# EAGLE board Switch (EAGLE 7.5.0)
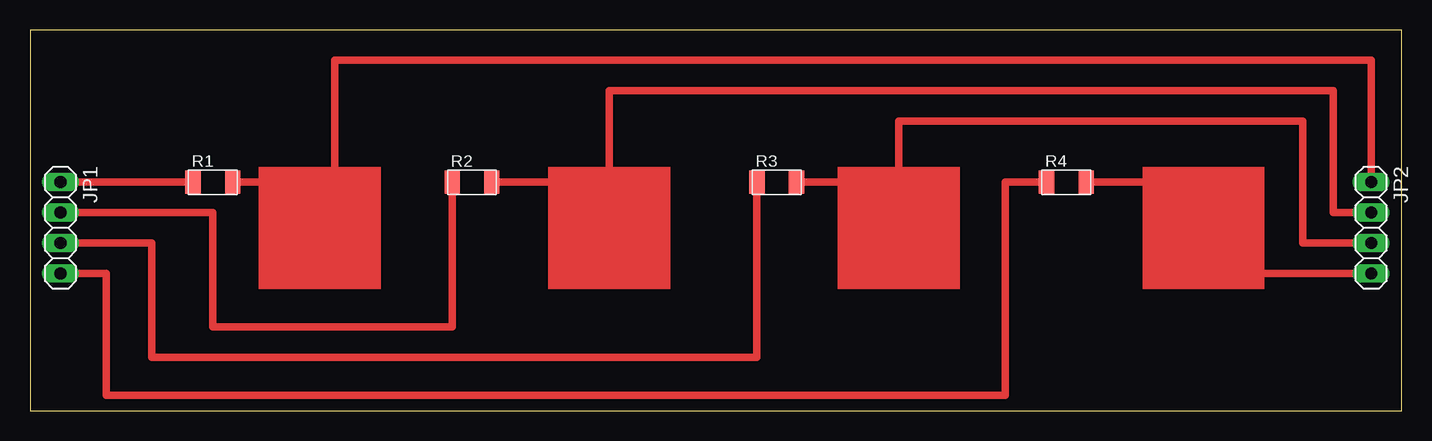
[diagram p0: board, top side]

Size 114.3 x 31.75 mm. Coordinates in mm from the lower left corner, seen from the top.
Outline: 0,0 114.3,0 114.3,31.75 0,31.75 0,0
Copper layers (1*16): Top 0.035mm / dielectric 1.5mm / Bottom 0.035mm
Design rules "default": minimum track width 10mil, minimum drill 24mil, track to track 8mil, track to pad 8mil, pad to pad 8mil, via to via 8mil, smd to smd 8mil, copper to edge 40mil, drill to drill 8mil, minimum pad ring 10mil, minimum via ring 8mil, stop-mask expansion 4mil, vias tented up to drill 0mil, thermal gap 10mil

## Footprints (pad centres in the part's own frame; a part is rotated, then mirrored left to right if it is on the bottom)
1X04 = drill 1.016 long: 1 -3.81,0; 2 -1.27,0; 3 1.27,0; 4 3.81,0
R1206FAB = smd 1.27 x 1.905: 1 -1.651,0; 2 1.651,0

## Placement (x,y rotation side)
JP1  [1X04]  2.54,15.24 270 top
JP2  [1X04]  111.76,15.24 270 top
R1  [R1206FAB]  15.24,19.05 0 top
R2  [R1206FAB]  36.83,19.05 0 top
R3  [R1206FAB]  62.23,19.05 0 top
R4  [R1206FAB]  86.36,19.05 0 top

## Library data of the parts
JP1 JP2 = pinhead
R1-R4 = fab

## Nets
N$1: JP1.1 R1.1
N$3: JP1.2 R2.1
N$4: JP2.2 R2.2
N$5: JP1.3 R3.1
N$6: JP2.3 R3.2
N$7: JP1.4 R4.1
N$8: JP2.4 R4.2
N$9: JP2.1 R1.2

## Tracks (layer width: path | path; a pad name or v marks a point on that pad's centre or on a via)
N$1
  Top 0.61: JP1.1 R1.1
N$3
  Top 0.61: JP1.2 15.24,16.51 15.24,6.99 35.18,6.99 R2.1
N$4
  Top 0.61: R2.2 48.26,19.05 48.26,26.67 108.58,26.67 108.58,16.51 JP2.2
N$5
  Top 0.61: JP1.3 10.16,13.97 10.16,4.45 60.58,4.45 R3.1
N$6
  Top 0.61: R3.2 72.39,19.05 72.39,24.13 106.05,24.13 106.05,13.97 JP2.3
N$7
  Top 0.61: JP1.4 6.35,11.43 6.35,1.27 81.28,1.27 81.28,19.05 R4.1
N$8
  Top 0.406: 99.06,19.05 99.06,11.43
  Top 0.61: R4.2 99.06,19.05 | 99.06,11.43 JP2.4
N$9
  Top 0.61: R1.2 25.4,19.05 25.4,29.21 111.76,29.21 JP2.1
(copper drawn outside any net)
  shapes: Top area x4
